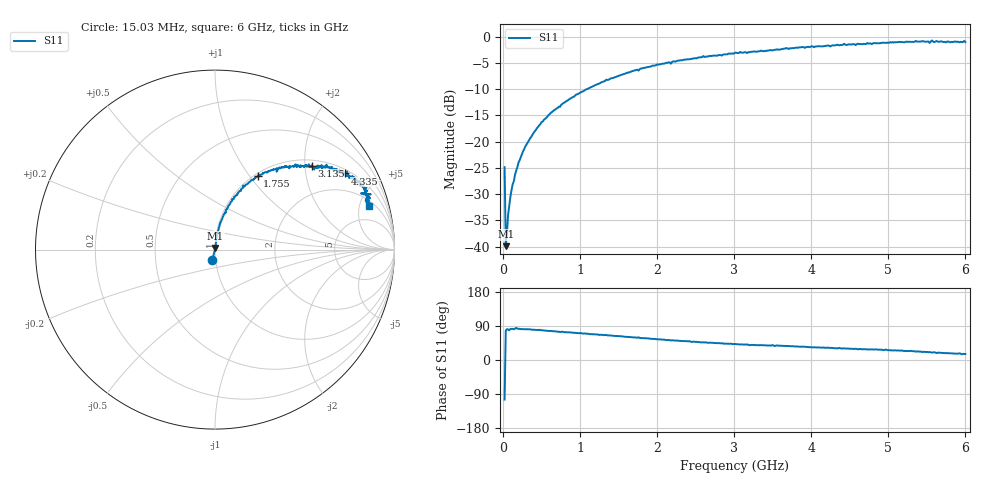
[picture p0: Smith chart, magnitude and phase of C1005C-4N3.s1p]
!	Network	Analyzer	HP8753E.07.74:	Oct	30	2002	Serial	No.	JP38451487
!	Hewlett-Packard
!	7	Sep	2009	8:24:16
!	Frequency	S11
#	HZ	S	RI	R	50
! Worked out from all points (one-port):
!   400 points, 15.03 MHz to 6 GHz, reference 50 ohm
!   lowest |S11| = -39.9 dB at 30.03 MHz (marker M1), VSWR 1.02, Z = 50.2 + j0.988 ohm
!   |S11| at or under -10 dB: start of sweep to 1.083 GHz
!   S11 on the Smith chart (normalised r, x): 15.03 MHz: 0.97, -0.11; 1.755 GHz: 1.03, +1.10; 3.135 GHz: 1.14, +2.16; 4.335 GHz: 1.16, +3.31; 6 GHz: 2.62, +6.13
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1.502992e7  -0.0143 -0.0553
3.002985e7  0.00225 0.00984
4.502978e7  0.00199 0.0131
6.00297e7  0.00323 0.0197
9.002955e7  0.00416 0.0294
1.200294e8  0.00534 0.039
1.95029e8  0.0081 0.0624
2.850286e8  0.0138 0.0894
4.350278e8  0.0255 0.132
7.650262e8  0.0605 0.221
1.065025e9  0.107 0.294
1.515022e9  0.197 0.38
1.755021e9  0.238 0.411
2.265019e9  0.371 0.461
3.015015e9  0.523 0.475
3.135014e9  0.538 0.468
3.765011e9  0.626 0.461
4.335008e9  0.723 0.424
4.515007e9  0.733 0.414
4.965005e9  0.773 0.404
5.265004e9  0.821 0.357
5.445003e9  0.848 0.326
5.520002e9  0.843 0.315
5.535002e9  0.813 0.313
5.565002e9  0.868 0.308
5.595002e9  0.831 0.31
5.625002e9  0.864 0.286
6e9  0.857 0.242
